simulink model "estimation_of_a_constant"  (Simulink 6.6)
settings: Solver=FixedStepDiscrete  StartTime=0.0  StopTime=499  FixedStep=1  RelTol=1e-3
libraries: simulink x2

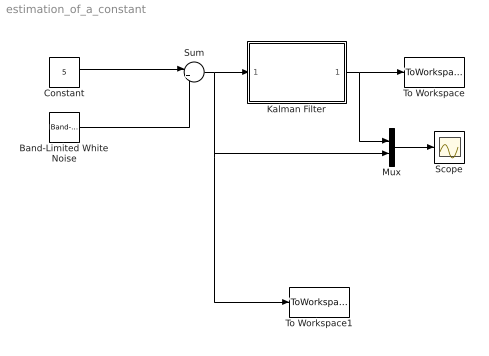
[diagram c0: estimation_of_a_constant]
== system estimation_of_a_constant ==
  Band-Limited White Noise : simulink/Sources/Band-Limited White Noise  SystemSampleTime=-1  Cov=[5]  Ts=1  seed=[23341]
  Constant : Constant  Value=5
  Kalman Filter : Subsystem  mask{timelimit=1000}
      mask prompts: timelimit "Time Limit"
  Mux : Mux  Inputs=2
  Scope : Scope
  Sum : Sum  Inputs=|++
  To Workspace : ToWorkspace  VariableName=simout  SampleTime=-1  SaveFormat=Array
  To Workspace1 : ToWorkspace  VariableName=simout1  SampleTime=-1  SaveFormat=Array
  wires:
  Sum/1 -> Kalman Filter/1(input), Mux/2, To Workspace1/1
  Kalman Filter/1(filtered input) -> To Workspace/1, Mux/1
  Constant/1 -> Sum/1
  Band-Limited White Noise/1 -> Sum/2
  Mux/1 -> Scope/1

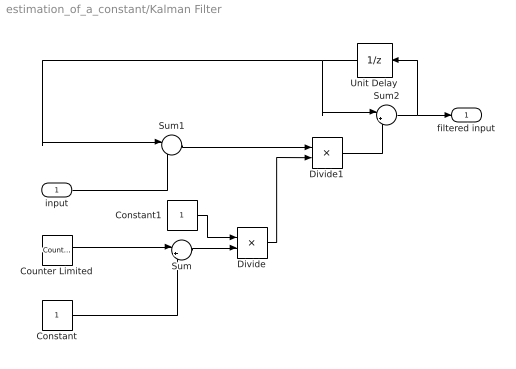
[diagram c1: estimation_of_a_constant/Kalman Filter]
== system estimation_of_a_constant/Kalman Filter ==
  input : Inport  SampleTime=1
  Constant : Constant  SampleTime=1
  Constant1 : Constant  SampleTime=1
  Counter Limited : simulink/Sources/Counter Limited  SystemSampleTime=-1  uplimit=timelimit  tsamp=1
  Divide : Product  Inputs=*/  OutScaling=2^-10  SampleTime=1
  Divide1 : Product  Inputs=**  OutScaling=2^-10  SampleTime=1
  Sum : Sum  Inputs=|++
  Sum1 : Sum  Inputs=|-+  SampleTime=1
  Sum2 : Sum  Inputs=|++  SampleTime=1
  Unit Delay : UnitDelay  Orientation=left
  filtered input : Outport  SampleTime=1
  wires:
  input/1 -> Sum1/2
  Sum1/1 -> Divide1/1
  Unit Delay/1 -> Sum2/1, Sum1/1
  Sum2/1 -> Unit Delay/1, filtered input/1
  Divide1/1 -> Sum2/2
  Divide/1 -> Divide1/2
  Constant1/1 -> Divide/1
  Sum/1 -> Divide/2
  Constant/1 -> Sum/2
  Counter Limited/1 -> Sum/1
